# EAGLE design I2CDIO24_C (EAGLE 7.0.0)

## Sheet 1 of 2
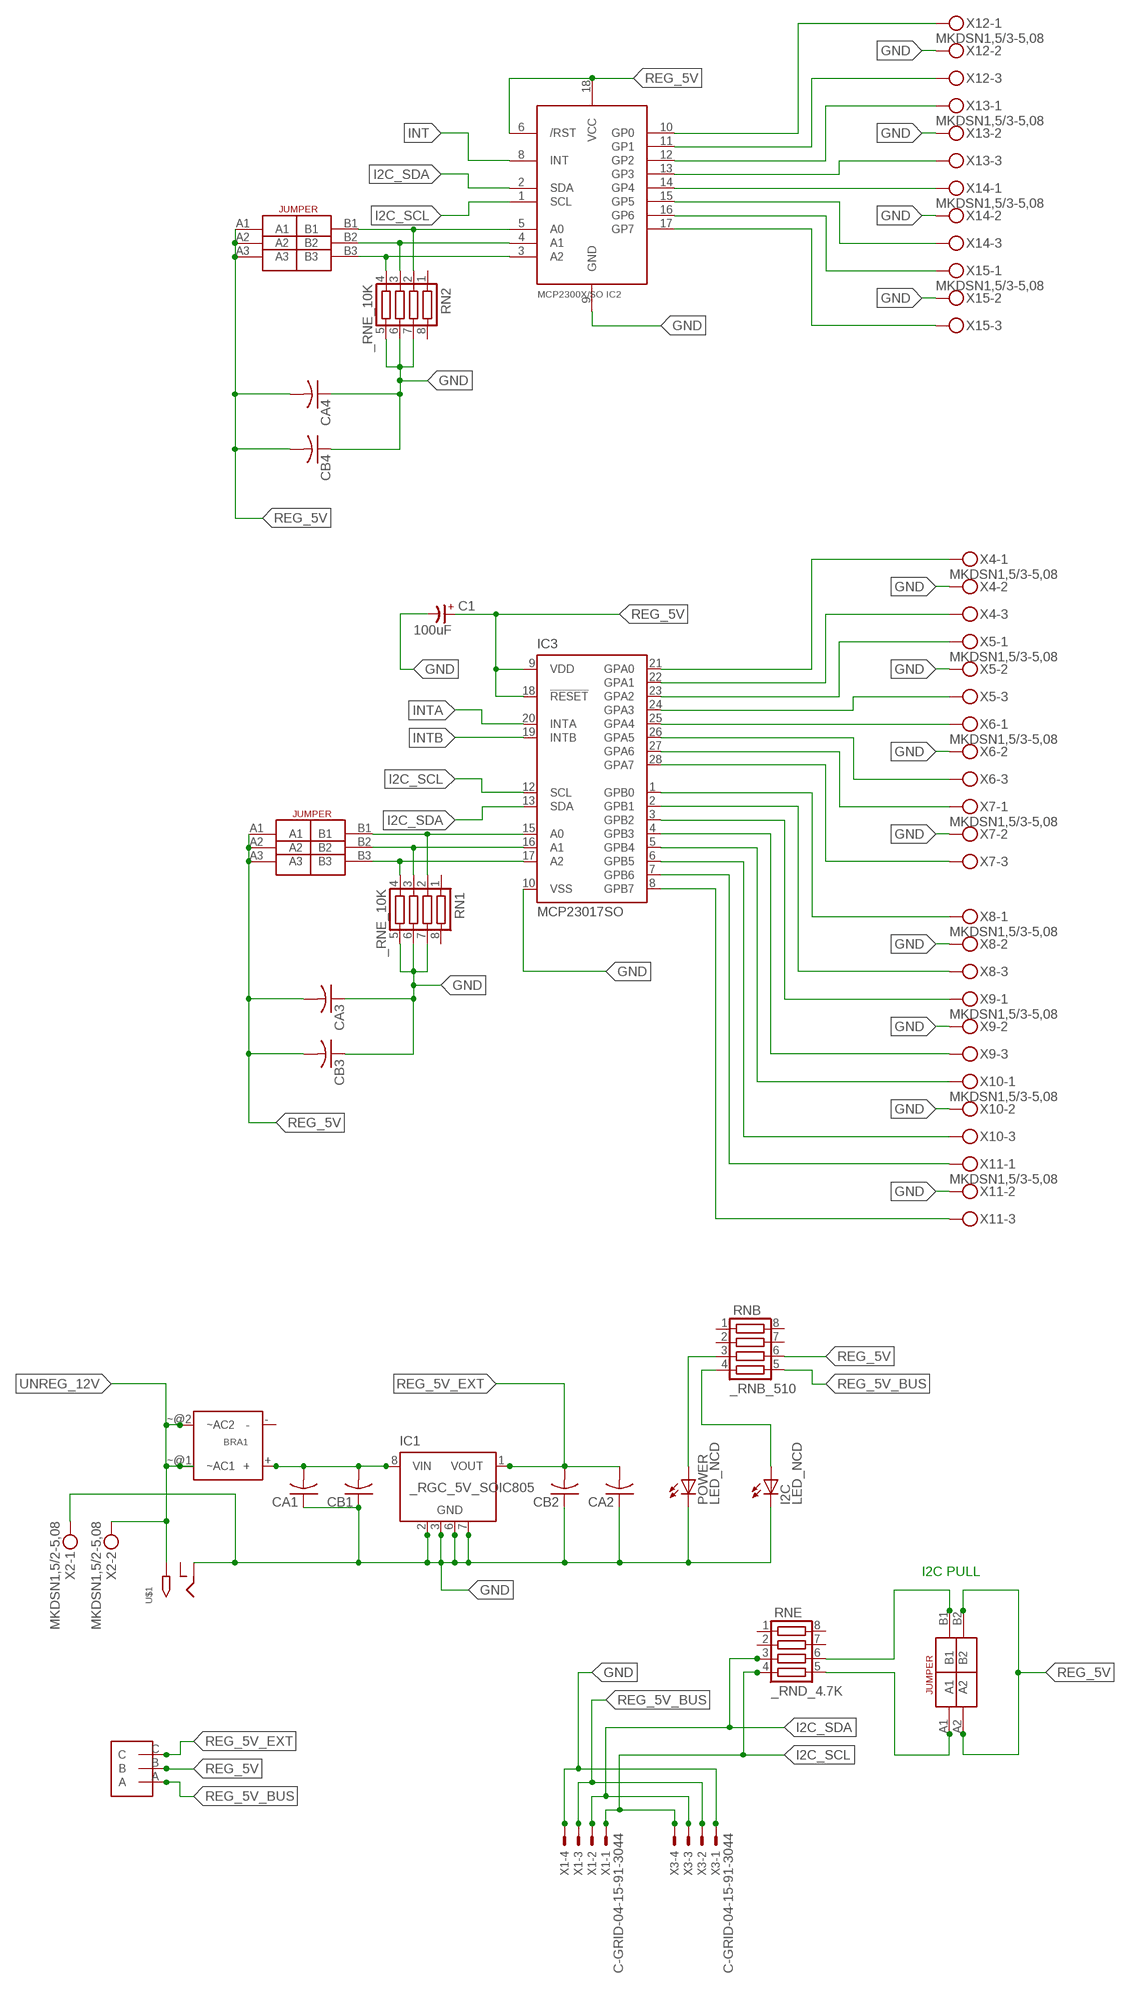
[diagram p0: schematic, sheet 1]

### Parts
BRA1  MB2S_  [MB2S]
C1  100uF  CP-E-025X060  [E-025X060]
CA1  CC1206KRX7R9BB104C1206K  [CC1206KRX7R9BB104]
CA2  CC1206KRX7R9BB104C1206K  [CC1206KRX7R9BB104]
CA3  CC1206KRX7R9BB104C1206K  [CC1206KRX7R9BB104]
CA4  CC1206KRX7R9BB104C1206K  [CC1206KRX7R9BB104]
CB1  TMK316F106ZL-TC1206K  [TMK316F106ZL-T]
CB2  TMK316F106ZL-TC1206K  [TMK316F106ZL-T]
CB3  TMK316F106ZL-TC1206K  [TMK316F106ZL-T]
CB4  TMK316F106ZL-TC1206K  [TMK316F106ZL-T]
I2C  LED_NCD  [CHIPLED_0603]
IC1  _RGC_5V_SOIC805  [_RGC_5V_SOIC8]
IC2  MCP2300X/SO  [SO18W]
IC3  MCP23017SO  [SO28W]
POWER  LED_NCD  [CHIPLED_0603]
RN1  _RNE_10K  [RNE]
RN2  _RNE_10K  [RNE]
RNB  _RNB_510  [RNB]
RNE  _RND_4.7K  [RND]
U$1  2.1MMJACK  [PJ-102A]
U$2  JUMPER_1X3  [JUMPER_1X3]
U$3  JUMPER_2X2  [JUMPER_2X2]
U$4  JUMPER_3X2  [JUMPER_3X2]
U$18  JUMPER_3X2  [JUMPER_3X2]
X1  C-GRID-04-15-91-3044  [15-91-04]
X2  MKDSN1,5/2-5,08  [MKDSN1,5/2-5,08]
X3  C-GRID-04-15-91-3044  [15-91-04]
X4  MKDSN1,5/3-5,08  [MKDSN1,5/3-5,08]
X5  MKDSN1,5/3-5,08  [MKDSN1,5/3-5,08]
X6  MKDSN1,5/3-5,08  [MKDSN1,5/3-5,08]
X7  MKDSN1,5/3-5,08  [MKDSN1,5/3-5,08]
X8  MKDSN1,5/3-5,08  [MKDSN1,5/3-5,08]
X9  MKDSN1,5/3-5,08  [MKDSN1,5/3-5,08]
X10  MKDSN1,5/3-5,08  [MKDSN1,5/3-5,08]
X11  MKDSN1,5/3-5,08  [MKDSN1,5/3-5,08]
X12  MKDSN1,5/3-5,08  [MKDSN1,5/3-5,08]
X13  MKDSN1,5/3-5,08  [MKDSN1,5/3-5,08]
X14  MKDSN1,5/3-5,08  [MKDSN1,5/3-5,08]
X15  MKDSN1,5/3-5,08  [MKDSN1,5/3-5,08]

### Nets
GND: C1.- CA1.1 CA2.1 CA3.1 CA4.1 CB1.1 CB2.1 CB3.1 CB4.1 I2C.C IC1.2(GND) IC1.3(GND) IC1.6(GND) IC1.7(GND) IC2.9(GND) IC3.10(VSS) POWER.C RN1.5 RN1.6 RN1.7 RN2.5 RN2.6 RN2.7 U$1.RING X1.4 X2.1 X3.1 X4.2 X5.2 X6.2 X7.2 X8.2 X9.2 X10.2 X11.2 X12.2 X13.2 X14.2 X15.2
I2C_SCL: IC2.1(SCL) IC3.12(SCL) RNE.4 X1.1 X3.4
I2C_SDA: IC2.2(SDA) IC3.13(SDA) RNE.3 X1.2 X3.3
INT: IC2.8(INT)
INTA: IC3.20(INTA)
INTB: IC3.19(INTB)
N$1: BRA1.+ CA1.2 CB1.2 IC1.8(VIN)
N$2: POWER.A RNB.3
N$3: I2C.A RNB.4
N$4: RNE.5 U$3.A1
N$5: RNE.6 U$3.B1
N$6: IC3.15(A0) RN1.2 U$18.B1
N$7: IC3.16(A1) RN1.3 U$18.B2
N$8: IC3.17(A2) RN1.4 U$18.B3
N$9: IC3.21(GPA0) X4.1
N$10: IC3.22(GPA1) X4.3
N$11: IC3.23(GPA2) X5.1
N$12: IC3.24(GPA3) X5.3
N$13: IC3.25(GPA4) X6.1
N$14: IC3.26(GPA5) X6.3
N$15: IC3.27(GPA6) X7.1
N$16: IC3.28(GPA7) X7.3
N$17: IC3.1(GPB0) X8.1
N$18: IC3.2(GPB1) X8.3
N$19: IC3.3(GPB2) X9.1
N$20: IC3.4(GPB3) X9.3
N$21: IC3.5(GPB4) X10.1
N$22: IC3.6(GPB5) X10.3
N$23: IC3.7(GPB6) X11.1
N$24: IC3.8(GPB7) X11.3
N$25: IC2.10(GP0) X12.1
N$26: IC2.11(GP1) X12.3
N$27: IC2.12(GP2) X13.1
N$28: IC2.13(GP3) X13.3
N$29: IC2.14(GP4) X14.1
N$30: IC2.15(GP5) X14.3
N$31: IC2.16(GP6) X15.1
N$32: IC2.17(GP7) X15.3
N$33: IC2.5(A0) RN2.2 U$4.B1
N$34: IC2.4(A1) RN2.3 U$4.B2
N$35: IC2.3(A2) RN2.4 U$4.B3
REG_5V: C1.+ CA3.2 CA4.2 CB3.2 CB4.2 IC2.6(/RST) IC2.18(VCC) IC3.9(VDD) IC3.18(!RESET) RNB.6 U$2.B U$3.A2 U$3.B2 U$4.A1 U$4.A2 U$4.A3 U$18.A1 U$18.A2 U$18.A3
REG_5V_BUS: RNB.5 U$2.A X1.3 X3.2
REG_5V_EXT: CA2.2 CB2.2 IC1.1(VOUT) U$2.C
UNREG_12V: BRA1.~@1(~AC1) BRA1.~@2(~AC2) U$1.TIP X2.2
Unconnected: BRA1.- IC1.4(NC) IC1.5(NC) RN1.1 RN1.8 RN2.1 RN2.8 RNB.1 RNB.2 RNB.7 RNB.8 RNE.1 RNE.2 RNE.7 RNE.8 U$1.RING_SW

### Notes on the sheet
- I2C PULL

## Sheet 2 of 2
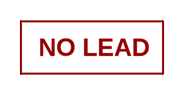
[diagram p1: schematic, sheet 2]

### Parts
U$16  NOPB_LOGO_SYM  [NOPB_LOGO_SYM]

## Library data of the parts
BRA1 = NCD_ULTIMATE_LIBRARY:MB2S: Bridge Rectifier BRA MB2S 200V 500ma Digikey MB2S-TPMSTR-ND/MB2S-TP
C1 = NCD_ULTIMATE_LIBRARY:CP-: Capacitors All Kinds POLARIZED CAP
CA1-CA4 = NCD_ULTIMATE_LIBRARY:CC1206KRX7R9BB104: Capacitor CA .1uF 50V SMT C1206K CC1206KRX7R9BB104
CB1-CB4 = NCD_ULTIMATE_LIBRARY:TMK316F106ZL-T: Capacitor CB 10uF SMT 1206 TMK316F106ZL-T
I2C POWER = NCD_ULTIMATE_bhaskar:LED_NCD
IC1 = NCD_ULTIMATE_LIBRARY:_RGC_5V_SOIC8: Regulator Linear 5V Chip Positive VOLTAGE REGULATOR Digikey 497-7267-2-ND/L78L05CD13TR
IC2 = NCD_ULTIMATE_LIBRARY:MCP2300X: Semiconductor Port Expander I/O 8-Bit I2C MCP23008 Inexpensive i2c i/o expander - 8 general purpose i/o pins with optional pullups
IC3 = NCD_ULTIMATE_LIBRARY:MCP23017: Semiconductor Port Expander I/O 16-Bit I2C http://ww1.microchip.com/downloads/en/DeviceDoc/21952a.pdf Source: http://ww1.microchip.com/downloads/en/DeviceDoc/21952a.pdf
RN1 RN2 = NCD_ULTIMATE_LIBRARY:_RNE_10K: Resistor Array RNE SMT 10K x 4 Single Resistor Source: http://www.ctscorp.com/components/Datasheets/CTSChipArrayDs.pdf Digikey 742C083103JPTR-ND/742C083103JP; OC_FARNELL: unknown; OC_NEWARK: unknown
RNB = NCD_ULTIMATE_LIBRARY:_RNB_510: Resistor Array RNB SMT 510 x 4 Single Resistor Source: http://www.ctscorp.com/components/Datasheets/CTSChipArrayDs.pdf Digikey 742C083511JPTR-ND/ 742C083511JP; OC_FARNELL: unknown; OC_NEWARK: unknown
RNE = NCD_ULTIMATE_LIBRARY:_RND_4.7K: Resistor Array RND SMT 4.7K x 4 Single Resistor Source: http://www.ctscorp.com/components/Datasheets/CTSChipArrayDs.pdf Digikey 742C083472JPTR-ND/742C083472JP; OC_FARNELL: unknown; OC_NEWARK: unknown
U$1 = NCD_ULTIMATE_CONNECTORS:2.1MMJACK: 2.1mm x 5.5mm DC jack with internal switch. Digikey part #PJ-102A, 4UCON part #05537 By microbuilder.eu
U$2 = NCD_ULTIMATE_CONNECTORS:JUMPER_1X3
U$3 = NCD_ULTIMATE_CONNECTORS:JUMPER_2X2
U$4 U$18 = NCD_ULTIMATE_CONNECTORS:JUMPER_3X2
U$16 = PatternAgents-Logos:NOPB_LOGO_SYM: NOPB_LOGO_SYM
X1 X3 = NCD_ULTIMATE_CONNECTORS:C-GRID-04: CONNECTOR 4-Pos I2C wire to board 2.54 mm (0.100") pitch header Digikey WM1342-ND/0015912045; OC_FARNELL: unknown; OC_NEWARK: unknown
X2 = NCD_ULTIMATE_CONNECTORS:MKDSN1,5/2-5,08: MKDSN 1,5/ 2-5,08 Printklemme
X4-X15 = NCD_ULTIMATE_CONNECTORS:MKDSN1,5/3-5,08: MKDSN 1,5/ 3-5,08 Printklemme Nennstrom: 13,5 A Nennspannung: 250 V Rastermaß: 5,08 mm Polzahl: 3 Anschlussart: Schraubanschluss Montage: Löten Anschlussrichtung Leiter/Platine: 0 ° Artikelnummer: 1729131 Source: http://eshop.phoenixcontact.com .. 1729131.pdf

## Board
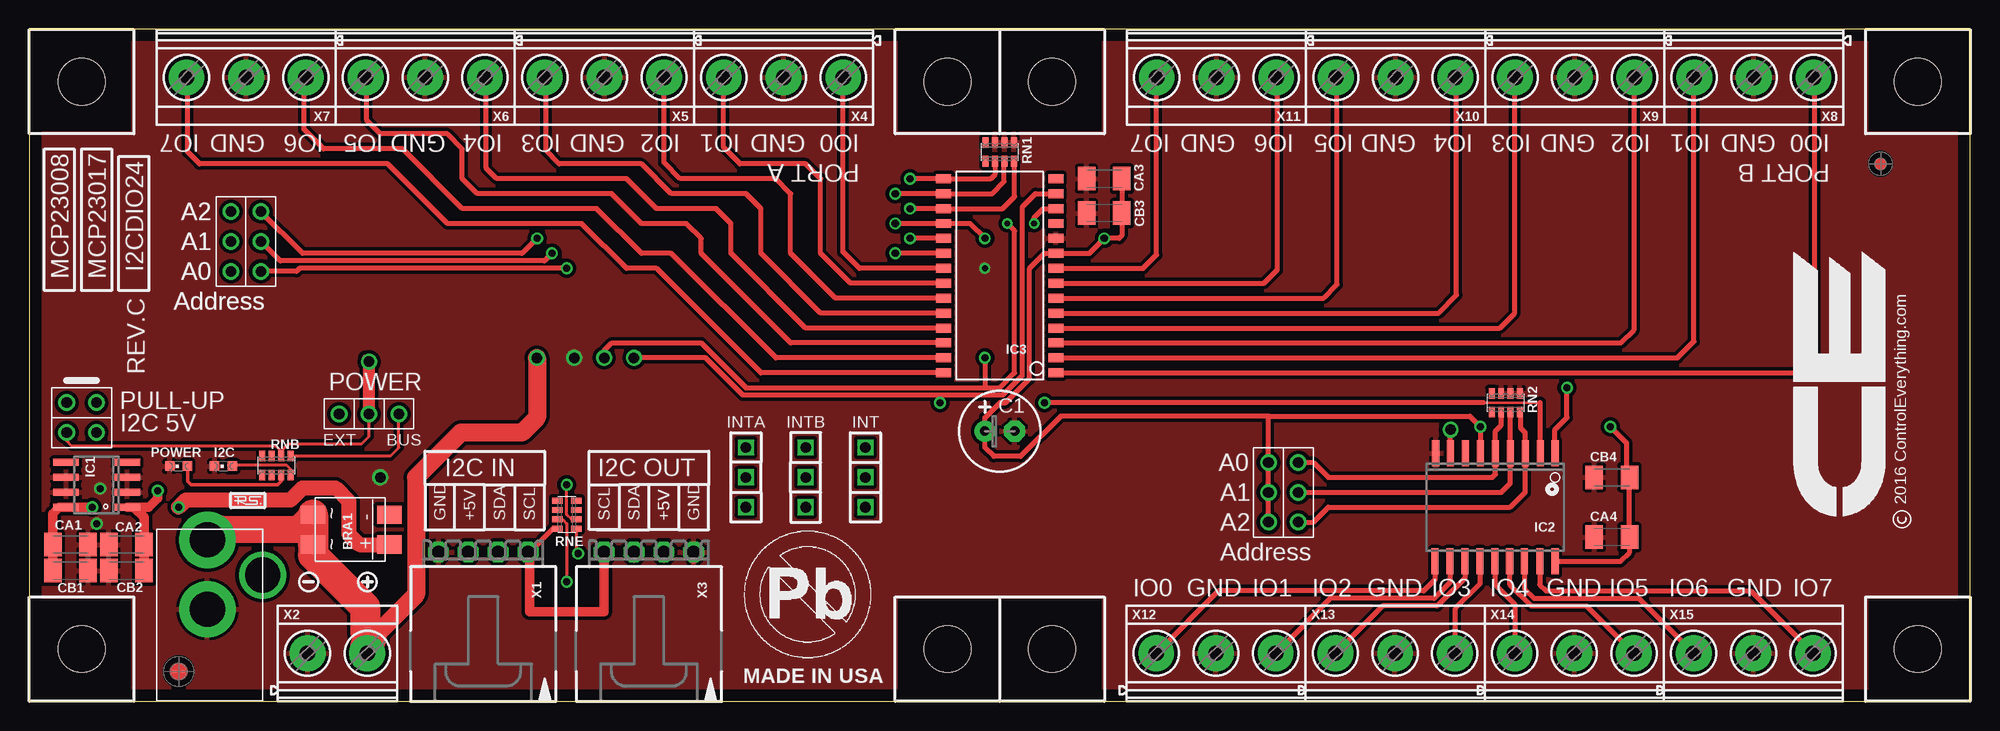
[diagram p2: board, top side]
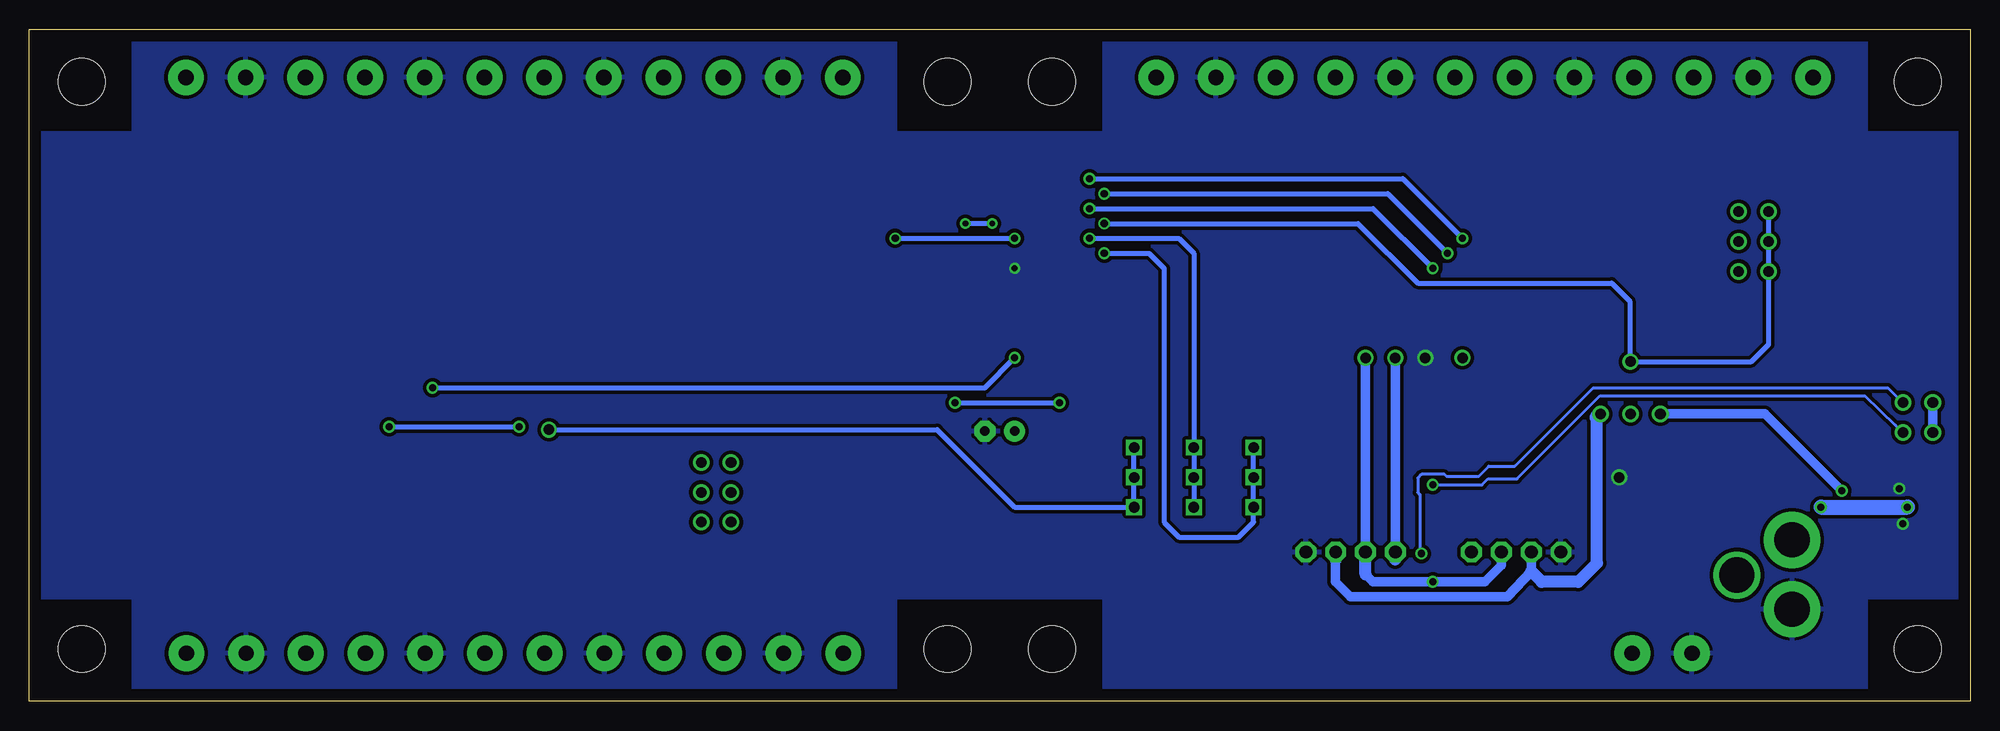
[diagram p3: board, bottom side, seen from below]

Size 165.1 x 57.15 mm. Coordinates in mm from the lower left corner, seen from the top.
Outline: 81.28,0 0,0 0,55.88
Outline: 81.28,0 82.53,0
Outline: 0,56.82 0,55.88
Outline: 81.28,0 82.55,0 163.83,0
Outline: 0,55.88 0,57.15 165.1,57.15 165.1,0 163.83,0
Outline: 163.83,0 165.08,0
Copper layers (1*16): Top 0.035mm / dielectric 1.5mm / Bottom 0.035mm
Design rules "default": minimum track width 10mil, minimum drill 24mil, track to track 8mil, track to pad 8mil, pad to pad 8mil, via to via 8mil, smd to smd 8mil, copper to edge 40mil, drill to drill 8mil, minimum pad ring 10mil, minimum via ring 8mil, stop-mask expansion 4mil, vias tented up to drill 0mil, thermal gap 10mil
Holes 3.96 mm at 4.45,4.45 78.11,4.45 78.11,52.7 4.45,52.7 78.11,52.7 87,52.7 87,4.45 160.66,4.45 160.66,52.7

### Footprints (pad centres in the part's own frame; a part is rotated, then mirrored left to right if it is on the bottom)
MB2S = smd 1.55 x 2.1: + 0,-6.5; - 2.54,-6.5; ~@1 0,0; ~@2 2.54,0
E-025X060 = drill 0.813 pad 1.778: + -1.27,0 | drill 0.813 pad 1.778 octagon: - 1.27,0
CC1206KRX7R9BB104 = smd 1.5 x 2: 1 -1.5,0; 2 1.5,0
TMK316F106ZL-T = smd 1.5 x 2: 1 -1.5,0; 2 1.5,0
CHIPLED_0603 = smd 0.8 x 0.8: A 0,-0.75; C 0,0.75
_RGC_5V_SOIC8 = smd 0.6 x 2.2: 1 -1.905,-2.6; 2 -0.635,-2.6; 3 0.635,-2.6; 4 1.905,-2.6; 5 1.905,2.6; 6 0.635,2.6; 7 -0.635,2.6; 8 -1.905,2.6
SO18W = smd 0.6 x 2.2: 1 -4.445,-4.6; 2 -3.175,-4.6; 3 -1.905,-4.6; 4 -0.635,-4.6; 5 0.635,-4.6; 6 1.905,-4.6; 7 3.175,-4.6; 8 4.445,-4.6; 9 5.715,-4.6; 10 5.775,4.6; 11 4.505,4.6; 12 3.235,4.6; 13 1.965,4.6; 14 0.695,4.6; 15 -0.575,4.6; 16 -1.845,4.6; 17 -3.145,4.6; 18 -4.445,4.6
SO28W = smd 0.762 x 1.27: 1 -7.62,-4.78; 2 -6.35,-4.78; 3 -5.08,-4.78; 4 -3.81,-4.78; 5 -2.54,-4.78; 6 -1.27,-4.78; 7 0,-4.78; 8 1.27,-4.78; 9 2.54,-4.78; 10 3.81,-4.78; 11 5.08,-4.78; 12 6.35,-4.78; 13 7.62,-4.78; 14 8.89,-4.78; 15 8.89,4.78; 16 7.62,4.78; 17 6.35,4.78; 18 5.08,4.78; 19 3.81,4.78; 20 2.54,4.78; 21 1.27,4.78; 22 0,4.78; 23 -1.27,4.78; 24 -2.54,4.78; 25 -3.81,4.78; 26 -5.08,4.78; 27 -6.35,4.78; 28 -7.62,4.78
RNE = smd 0.5 x 0.9: 1 -1.2,-0.8; 2 -0.4,-0.8; 3 0.4,-0.8; 4 1.2,-0.8; 5 1.2,0.8; 6 0.4,0.8; 7 -0.4,0.8; 8 -1.2,0.8
RNB = smd 0.5 x 0.9: 1 -1.2,-0.8; 2 -0.4,-0.8; 3 0.4,-0.8; 4 1.2,-0.8; 5 1.2,0.8; 6 0.4,0.8; 7 -0.4,0.8; 8 -1.2,0.8
RND = smd 0.5 x 0.9: 1 -1.2,-0.8; 2 -0.4,-0.8; 3 0.4,-0.8; 4 1.2,-0.8; 5 1.2,0.8; 6 0.4,0.8; 7 -0.4,0.8; 8 -1.2,0.8
PJ-102A = drill 3 pad 4.8: RING 0.1,-3.39; TIP 0.1,-9.29 | drill 3 pad 3.251: RING_SW -4.6,-6.29
JUMPER_1X3 = drill 0.9: A 0,5.08; B 0,2.54; C 0,0
JUMPER_2X2 = drill 0.9: A1 0,2.54; A2 0,0; B1 2.54,2.54; B2 2.54,0
JUMPER_3X2 = drill 0.9: A1 0,5.08; A2 0,2.54; A3 0,0; B1 2.54,5.08; B2 2.54,2.54; B3 2.54,0
15-91-04 = drill 1.1 pad 1.778 octagon: 1 -3.81,-7.62; 2 -1.27,-7.62; 3 1.27,-7.62; 4 3.81,-7.62
MKDSN1,5/2-5,08 = drill 1.3 pad 3.048: 1 -2.561,0.025; 2 2.519,0.025
MKDSN1,5/3-5,08 = drill 1.3 pad 3.048: 1 -7.641,0.025; 2 -2.561,0.025; 3 2.519,0.025

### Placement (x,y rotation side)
BRA1  24.13,13.34 90 top
C1  82.55,22.99 0 top
CA1  3.49,13.34 180 top
CA2  8.26,13.34 0 top
CA3  91.44,44.45 0 top
CA4  134.62,13.97 0 top
CB1  3.49,11.11 180 top
CB2  8.26,11.11 0 top
CB3  91.44,41.53 0 top
CB4  134.62,19.05 0 top
I2C  16.51,20 90 top
IC1  5.71,18.41 90 top
IC2  125.35,16.51 180 top
IC3  82.55,35.56 90 top
POWER  12.7,20 90 top
RN1  82.55,46.74 0 top
RN2  125.6,25.4 0 top
RNB  21.02,20.07 0 top
RNE  45.72,15.88 270 top
U$1  15.24,4.45 180 top
U$2  26.35,24.45 270 top
U$3  3.17,25.4 270 top
U$4  105.41,15.24 0 top
U$10  [VISION_REF15]  12.7,2.54 0 top
U$16  60.6,3.25 0 top
U$18  17.14,36.58 0 top
U$19  [VISION_REF10]  157.48,45.72 0 top
U$21  [ICON_USA]  60.71,1.52 0 top
U$22  [ICON_MINUS]  23.75,10.16 180 top
U$24  [ICON_PLUS]  28.77,10.16 90 top
X1  38.61,5.08 180 top
X2  26.23,4.06 0 top
X3  52.7,5.08 180 top
X4  61.59,53.09 180 top
X5  46.35,53.09 180 top
X6  31.11,53.09 180 top
X7  15.88,53.09 180 top
X8  144.15,53.09 180 top
X9  128.91,53.09 180 top
X10  113.67,53.09 180 top
X11  98.42,53.09 180 top
X12  103.5,4.06 0 top
X13  118.75,4.06 0 top
X14  133.99,4.06 0 top
X15  149.22,4.06 0 top

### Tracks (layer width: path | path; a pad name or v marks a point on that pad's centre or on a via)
GND  (via drill 0.5, 0.6, 0.9)
  Top 0.406: 34.8,12.38 X1.4
  Top 0.813: X3.1 56.52,12.06
  other vias: 5.71,15.11 6.03,18.1 46.35,29.21 29.84,19.05 81.28,36.83
  pour Bottom (isolate 0.305): -0.64,8.89 -0.64,48.26 8.89,48.26 8.89,57.78 73.66,57.78 73.66,48.26 91.44,48.26 91.44,57.78 156.21,57.78 156.21,48.26 165.74,48.26 165.74,8.89 156.21,8.89 156.21,-0.64 91.44,-0.64 91.44,8.89 73.66,8.89 73.66,-0.64 8.89,-0.64 8.89,8.89
  pour Top (isolate 0.305): -2.54,48.26 8.89,48.26 8.89,59.05 73.66,59.05 73.66,48.26 91.44,48.26 91.44,59.05 156.21,59.05 156.21,48.26 168.28,48.26 168.28,8.89 156.21,8.89 156.21,-2.54 91.44,-2.54 91.44,8.89 73.66,8.89 73.66,-2.54 8.89,-2.54 8.89,8.89 -1.91,8.89 -1.91,9.53 -2.54,9.53
I2C_SCL  (via drill 0.5, 0.6, 0.9)
  Top 0.406: RNE.4 44.51,14.68 42.55,12.7 | v48.9,29.21 48.9,29.84 49.53,30.48 57.15,30.48 60.96,26.67 81.28,26.67 | 81.28,26.67 82.55,26.67 83.82,27.94 83.82,40.01 v83.19,40.64 | IC2.1 129.79,23.11 130.81,24.13 v130.81,26.67 | v81.28,29.21 81.28,26.67 | v85.47,40.64 85.47,41.15 86.23,41.91 IC3.12
  Top 0.813: X3.4 48.9,7.62 42.55,7.62 42.55,12.7 X1.1
  Bottom 0.406: v130.81,26.67 83.82,26.67 v81.28,29.21 | v83.19,40.64 v85.47,40.64
  Bottom 0.813: v48.9,29.21 X3.4
  Bottom 1.016: 48.9,12.06 X3.4
I2C_SDA  (via drill 0.6, 0.9)
  Top 0.229: 128.52,25.4 123.7,25.4
  Top 0.254: RNE.3 45.36,15.47 45.72,15.11 v45.72,10.16
  Top 0.406: 77.47,26.04 82.8,26.04 84.45,27.69 84.45,42.04 85.6,43.18 IC3.13 | 77.47,26.04 60.71,26.04 57.53,29.21 v51.44,29.21 | IC2.2 128.52,25.4 | 123.7,25.4 v86.36,25.4 | v77.47,25.4 77.47,26.04
  Top 0.61: X3.3 51.44,12.06 | X1.2 39.88,12.38
  Bottom 0.406: v86.36,25.4 v77.47,25.4
  Bottom 0.813: 39.88,12.38 39.88,11.56 41.27,10.16 v45.72,10.16 50.8,10.16 51.44,10.79 | X3.3 v51.44,29.21
  Bottom 1.016: 39.88,12.38 X1.2 | 51.44,10.79 X3.3
INT  (via drill 0.9)
  Top 0.406: IC2.8 v120.9,23.11
  Bottom 0.406: v120.9,23.11 87.88,23.11 81.28,16.51 v71.12,16.51 v71.12,19.05 v71.12,21.59
INTA  (via drill 0.6, 0.9)
  Top 0.406: IC3.20 v73.66,38.1
  Bottom 0.406: v73.66,38.1 69.85,38.1 68.58,36.83 68.58,15.24 67.31,13.97 62.23,13.97 60.96,15.24 v60.96,16.51 v60.96,19.05 v60.96,21.59
INTB  (via drill 0.6, 0.9)
  Top 0.406: IC3.19 v74.93,39.37
  Bottom 0.406: v74.93,39.37 67.31,39.37 66.04,38.1 v66.04,21.59 v66.04,19.05 v66.04,16.51
N$1  (via drill 0.6)
  Top 0.813: CB1.2 CA1.2 1.99,15.96 2.54,16.51 IC1.8 v5.33,16.51
  Top 1.27: v12.7,16.51 13.34,17.14 22.23,17.14 23.24,18.16 26.04,18.16 27.18,17.02 27.18,14.22 28.07,13.34 BRA1.+
  Bottom 1.27: v12.7,16.51 v5.33,16.51
N$2
  Top 0.305: RNB.3 21.4,18.95 21.4,18.7 21.12,18.41 13.78,18.41 13.45,18.74 POWER.A
N$3
  Top 0.254: 22.23,18.95 22.23,19.74 21.9,20.07 16.94,20.07
  Top 0.305: RNB.4 22.23,18.95 | 16.94,20.07 I2C.A
N$4  (via drill 0.6)
  Top 0.254: RNE.5 46.52,12.6 v46.67,12.57
  Bottom 0.254: U$3.A1 6.99,26.67 32.07,26.67 38.73,20 40.96,20 41.85,19.11 44.51,19.11 44.7,19.3 46.67,19.3 46.99,18.99 46.99,17.78 46.8,17.59 46.8,12.7 v46.67,12.57
N$5  (via drill 0.6)
  Top 0.254: RNE.6 46.12,15.47 45.72,15.88 v45.72,18.41
  Bottom 0.254: v45.72,18.41 41.53,18.41 41.02,18.92 38.54,18.92 31.5,25.97 8.95,25.97 6.35,23.5 U$3.B1
N$6  (via drill 0.6)
  Top 0.406: RN1.2 82.17,45.92 82.17,44.83 81.79,44.45 IC3.15 v74.93,44.45 | v43.18,39.37 41.91,38.1 23.24,38.1 U$18.B1
  Bottom 0.406: v74.93,44.45 48.26,44.45 v43.18,39.37
N$7  (via drill 0.6)
  Top 0.406: RN1.3 82.93,45.92 82.93,44.2 81.92,43.18 IC3.16 v73.66,43.18 | v44.45,38.1 43.81,37.47 21.34,37.47 U$18.B2
  Bottom 0.406: v73.66,43.18 49.53,43.18 v44.45,38.1
N$8  (via drill 0.6)
  Top 0.406: RN1.4 83.82,45.87 83.82,42.93 82.8,41.91 IC3.17 v74.93,41.91 | v45.72,36.83 22.99,36.83 22.73,36.58 U$18.B3
  Bottom 0.406: v74.93,41.91 50.8,41.91 v45.72,36.83
N$9
  Top 0.406: IC3.21 70.61,36.83 69.22,38.23 69.22,53.04 X4.1
N$10
  Top 0.406: IC3.22 69.85,35.56 67.31,38.1 67.31,44.45 66.04,45.72 60.45,45.72 59.05,47.12 59.05,53.04 X4.3
N$11
  Top 0.406: IC3.23 68.58,34.29 64.77,38.1 64.77,43.18 63.5,44.45 55.37,44.45 53.98,45.85 53.98,53.04 X5.1
N$12
  Top 0.406: IC3.24 67.31,33.02 62.23,38.1 62.23,41.91 60.96,43.18 54.61,43.18 52.07,45.72 45.09,45.72 43.94,46.86 43.94,52.95 X5.3
N$13
  Top 0.406: IC3.25 66.04,31.75 59.69,38.1 59.69,40.64 58.42,41.91 53.34,41.91 50.8,44.45 39.75,44.45 38.86,45.34 38.86,52.95 X6.1
N$14
  Top 0.406: IC3.26 64.77,30.48 57.15,38.1 57.15,39.37 55.88,40.64 52.07,40.64 49.53,43.18 38.1,43.18 36.83,44.45 36.83,46.99 35.56,48.26 29.84,48.26 28.7,49.4 28.7,52.95 X6.3
N$15
  Top 0.406: IC3.27 63.5,29.21 54.61,38.1 52.07,38.1 48.26,41.91 36.83,41.91 31.75,46.99 25.02,46.99 23.37,48.64 23.37,52.91 X7.1
N$16
  Top 0.406: IC3.28 62.23,27.94 53.34,36.83 50.8,36.83 46.99,40.64 35.56,40.64 30.48,45.72 14.48,45.72 13.46,46.74 13.46,52.95 X7.3
N$17
  Top 0.406: IC3.1 150.75,27.94 151.89,29.08 151.89,52.95 X8.1
N$18
  Top 0.406: IC3.2 140.21,29.21 141.6,30.61 141.6,53.04 X8.3
N$19
  Top 0.406: IC3.3 135.38,30.48 136.53,31.62 136.53,53.04 X9.1
N$20
  Top 0.406: IC3.4 125.09,31.75 126.36,33.02 126.36,53.04 X9.3
N$21
  Top 0.406: IC3.5 119.89,33.02 121.41,34.54 121.41,52.95 X10.1
N$22
  Top 0.406: IC3.6 110.11,34.29 111.25,35.43 111.25,52.95 X10.3
N$23
  Top 0.406: IC3.7 105.03,35.56 106.17,36.7 106.17,52.95 X11.1
N$24
  Top 0.406: IC3.8 94.74,36.83 95.89,37.97 95.89,53.04 X11.3
N$25
  Top 0.406: IC2.10 119.57,10.35 118.62,9.4 101.17,9.4 X12.1
N$26
  Top 0.406: IC2.11 120.84,10.1 119.51,8.76 110.7,8.76 X12.3
N$27
  Top 0.406: IC2.12 122.11,10.48 119.76,8.13 115.14,8.13 X13.1
N$28
  Top 0.406: IC2.13 123.38,9.97 121.28,7.87 121.28,4.11 X13.3
N$29
  Top 0.406: IC2.14 124.65,9.97 126.36,8.26 126.36,4.11 X14.1
N$30
  Top 0.406: IC2.15 125.92,9.97 127.76,8.13 132.47,8.13 X14.3
N$31
  Top 0.406: IC2.16 127.19,9.59 128.02,8.76 136.91,8.76 X15.1
N$32
  Top 0.406: IC2.17 128.49,9.94 129.03,9.4 146.44,9.4 X15.3
N$33
  Top 0.406: U$4.B1 109.22,20.32 110.49,19.05 124.46,19.05 124.71,19.3 IC2.5 124.71,22.99 125.22,23.5 125.22,24.58 RN2.2
N$34
  Top 0.406: U$4.B2 125.22,17.78 125.98,18.54 IC2.4 125.98,24.58 RN2.3
N$35
  Top 0.406: RN2.4 126.87,24.53 126.87,23.24 127.25,22.86 IC2.3 127.25,17.78 125.98,16.51 110.49,16.51 109.22,15.24 U$4.B3
REG_5V  (via drill 0.6, 0.9)
  Top 0.254: RNB.6 21.42,21.29 | 21.42,21.29 22.04,21.91 28.26,21.91 28.89,22.54 U$2.B | 21.42,21.29 20.99,21.72 3.62,21.72 3.17,22.16 U$3.B2
  Top 0.406: v134.49,23.37 135.89,21.97 135.89,19.05 CB4.2 CA4.2 136.14,13.95 136.14,12.7 135.35,11.91 IC2.18 | v81.28,39.37 80.01,40.64 IC3.18 v73.66,40.64 | CA3.2 CB3.2 92.94,39.6 92.71,39.37 v91.44,39.37 90.17,38.1 IC3.9 86.36,38.1 85.09,36.83 85.09,27.43 83.06,25.4 82.55,25.4 81.28,24.13 C1.+ 81.28,21.59 82.04,20.83 84.33,20.83 87.76,24.26 105.41,24.26 | IC2.6 v123.44,23.37 122.56,24.26 105.41,24.26 | U$4.A3 U$4.A2 U$4.A1 105.41,24.26
  Top 0.61: 28.57,29.21 v28.89,28.89
  Top 1.016: U$2.B v28.89,28.89
  Bottom 0.406: 28.7,29.08 v28.89,28.89 | v91.44,39.37 v81.28,39.37 | v28.89,28.89 18.61,28.89 17.14,30.35 U$18.A3 U$18.A2 U$18.A1 | v73.66,40.64 52.07,40.64 46.99,35.56 30.48,35.56 28.96,34.04 28.96,28.96 v28.89,28.89 | v134.49,23.37 v123.44,23.37
  Bottom 0.813: U$3.B2 U$3.A2
REG_5V_BUS
  Top 0.254: U$2.A 31.43,21.59 30.71,20.87 RNB.5
  Top 0.61: X1.3 37.34,12.38 | X3.2 53.98,12.06
  Bottom 0.813: 37.34,12.38 37.34,11.05 39.37,8.89 52.7,8.89 53.98,10.16 53.98,12.06
  Bottom 1.016: 31.75,24.13 31.75,11.75 33.34,10.16 36.45,10.16 37.34,11.05 | 37.34,12.38 X1.3 | 53.98,12.06 X3.2
  Bottom 1.27: 31.75,24.13 U$2.A
REG_5V_EXT  (via drill 0.6)
  Top 0.813: CB2.2 CA2.2 9.76,15.64 8.89,16.51 | 8.89,16.51 IC1.1 | v10.92,17.91 10.92,17.27 10.16,16.51 8.89,16.51
  Bottom 0.813: v10.92,17.91 17.46,24.45 U$2.C
UNREG_12V  (via drill 0.9)
  Top 1.524: v43.18,29.21 43.18,24.13 41.91,22.86 36.7,22.86 32.89,19.05 32.89,9.08 29.11,5.3 28.57,4.76
  Top 2.286: BRA1.~@2 22.86,14.61 16.01,14.61
  Top 2.54: 16.01,14.61 U$1.TIP | X2.2 28.55,4.45 28.57,4.76 | BRA1.~@2 BRA1.~@1 24.13,12.45 28.57,8 28.57,5.84 29.11,5.3

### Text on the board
tNames: IO7 | GND | IO6 | IO5 | GND | IO4 | IO3 | GND | IO2 | IO1 | GND | IO0 | IO7 | GND | IO6 | IO5 | GND | IO4 | IO3 | GND | IO2 | IO1 | GND | IO0 | MCP23008 | MCP23017 | I2CDIO24 | PORT A | PORT B | A2 | A2 | A1 | A1 | A0 | A0 | REV.C | Address | Address | POWER | PULL-UP | I2C 5V | INTA | INTB | INT | EXT | BUS | A0 | I2C IN | I2C OUT | A1 | 2016 ControlEverything.com | GND | +5V | SDA | SCL | SCL | SDA | +5V | +5V | GND | A2 | Address | IO0 | GND | IO1 | IO2 | GND | IO3 | IO4 | GND | IO5 | IO6 | GND | IO7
